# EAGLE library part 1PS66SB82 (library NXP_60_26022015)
15 V, 30 mA low Cd Schottky barrier diode Epitaxial low capacitance Schottky barrier diodes encapsulated in very small SMD plastic packages. AAL Eindhoven MK
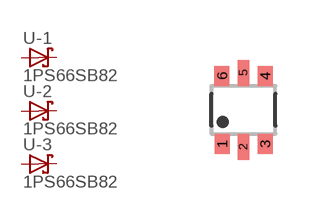
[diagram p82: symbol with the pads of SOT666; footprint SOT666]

Designator prefix -; gates -1=DIODE_SCHOTTKY -2=DIODE_SCHOTTKY -3=DIODE_SCHOTTKY

## 1PS66SB82  [SOT666]
1  -1:A  pas
2  -2:A  pas
3  -3:A  pas
4  -3:K  pas
5  -2:K  pas
6  -1:K  pas

## Footprint SOT666 (pad centres in mm)
SOT 666 Reflow soldering foorprint Source: Philips - BAS70_1PS7XSB70_SER_8.pdf
smd 0.375 x 0.5: 1 -0.537,-0.85; 3 0.538,-0.85; 4 0.538,0.85; 6 -0.538,0.85
smd 0.3 x 0.65: 2 0,-0.925; 5 0,0.925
